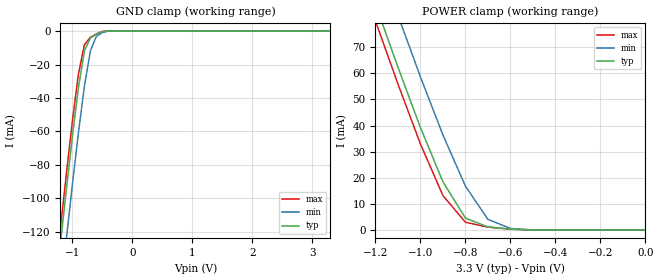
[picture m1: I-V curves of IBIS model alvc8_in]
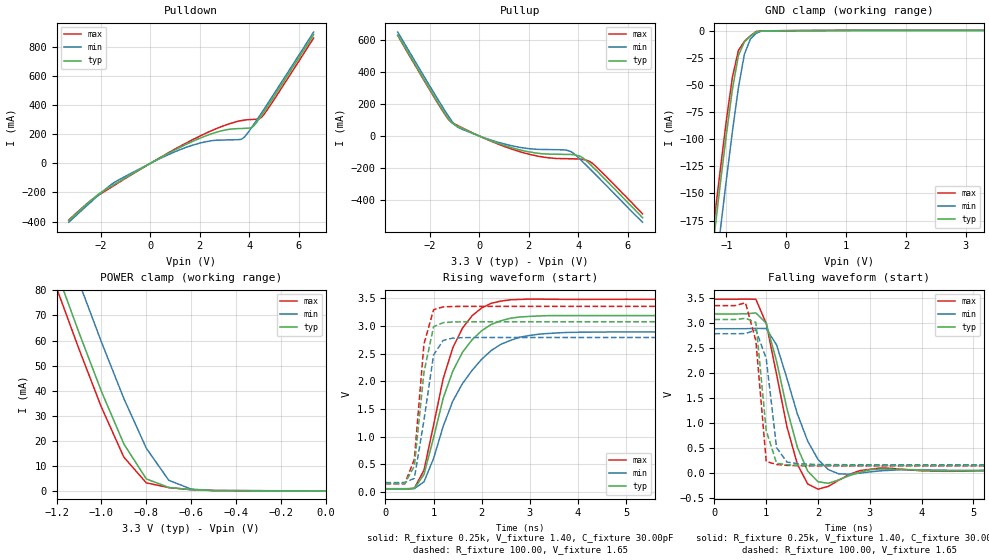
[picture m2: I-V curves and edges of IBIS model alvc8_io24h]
| IBIS file 16260ah.ibs created by s2ibis2 version 1.1
| North Carolina State University Electronics Research Laboratory  1995
[IBIS ver]   2.1
[File name]   16260ah.ibs
[File Rev]   1.0
[Date]   03/01/99 rtk rtk
[Source]   Integrated Device Technology, Inc.
[Notes]   1.Temperatures: typ=25C, min=100C, max=0C 2.RRmp rates based
   on 50 ohm load.
[Disclaimer] Integrated Device Technology, Inc. ("IDT") hereby grants the
   user of this IBIS model a non-exclusive, nontransferable
   license to use this IBIS model under the following terms. The
   user is granted this license only to use the IBIS model and is
   not granted rights to sell, copy (except as needed to run the
   IBIS model), rent, lease or sub-license the IBIS model in
   whole or in part, or in modified form to anyone. The User may
   modify the IBIS model to suit its specific applications, but
   rights to derivative works and such modifications shall belong
   to IDT. This IBIS model is provided on an AS IS" basis and IDT
   makes absolutely no warranty with respect to the information
   contained herein. IDT DISCLAIMS AND CUSTOMER WAIVES ALL
   WARRANTIES, EXPRESS AND IMPLIED, INCLUDING WARRANTIES OF
   MERCHANTABILITY AND FITNESS FOR A PARTICULAR PURPOSE. THE
   ENTIRE RISK AS TO QUALITY AND PERFORMANCE IS WITH THE USER
   ACCORDINGLY, IN NO EVENT SHALL IDT BE LIABLE FOR ANY DIRECT OR
   INDIRECT DAMAGES, WHETHER IN CONTRACT OR TORT, INCLUDING ANY
   LOST PROFITS OR OTHER INCIDENTAL, CONSEQUENTIAL, EXEMPLARY, OR
   PUNITIVE DAMAGES ARISING OUT OF THE USE OR APPLICATION OF THE
   IBIS model. Further, IDT reserves the right to make changes
   without notice to any product herein to improve reliability,
   function, or design. IDT does not convey any license under
   patent rights or any other intellectual property rights,
   including those of third parties. IDT is not obligated to
   provide maintenance or support for the licensed IBIS model.
[Copyright]   Copyright 1997, Integrated Device Technology, Inc. all rights
   reserved
|   Component ALVCH16260
[Component]   ALVCH1620
[Manufacturer]   Integrated Device Technology
[Package]
| PA56
| variable   typ   min   max
R_pkg   6.50m   5.00m   10.00m
L_pkg   3.30nH   2.50nH   4.90nH
C_pkg   0.29pF   0.010pF   1.16pF
[Pin]  signal_name   model_name   R_pin   L_pin   C_pin
1   OEA_   alvc8_in
2   LE1B   alvc8_in
3   2B3   alvc8_io24h
4   GND   GND
5   2B2   alvc8_io24h
6   2B1   alvc8_io24h
7   VCC   POWER
8   A1   alvc8_io24h
9   A2   alvc8_io24h
10   A3   alvc8_io24h
11   GND   GND
12   A4   alvc8_io24h
13   A5   alvc8_io24h
14   A6   alvc8_io24h
15   A7   alvc8_io24h
16   A8   alvc8_io24h
17   A9   alvc8_io24h
18   GND   GND
19   A10   alvc8_io24h
20   A11   alvc8_io24h
21   A12   alvc8_io24h
22   VCC   POWER
23   1B1   alvc8_io24h
24   1B2   alvc8_io24h
25   GND   alvc8_io24h
26   1B3   alvc8_io24h
27   LE2B   alvc8_in
28   SEL   alvc8_in
29   OE1B_   alvc8_in
30   LEA1B   alvc8_in
31   1B4   alvc8_io24h
32   GND   GND
33   1B5   alvc8_io24h
34   1B6   alvc8_io24h
35   VCC   POWER
36   1B7   alvc8_io24h
37   1B8   alvc8_io24h
38   1B9   alvc8_io24h
39   GND   GND
40   1B10   alvc8_io24h
41   1B11   alvc8_io24h
42   1B12   alvc8_io24h
43   2B12   alvc8_io24h
44   2B11   alvc8_io24h
45   2B10   alvc8_io24h
46   GND   GND
47   2B9   alvc8_io24h
48   2B8   alvc8_io24h
49   2B7   alvc8_io24h
50   VCC   POWER
51   2B6   alvc8_io24h
52   2B5   alvc8_io24h
53   GND   GND
54   2B4   alvc8_io24h
55   LEA2B   alvc8_in
56   OE2B_   alvc8_in
| Models and submodels in the file (2): alvc8_in (Input), alvc8_io24h (I/O)
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| in   in   dummy_model
| oe   oe   dummy_model
|   Model alvc8_in
[Model]   alvc8_in
Model_type   Input
Vinl =  0.800V
Vinh =  2.000V
C_comp   3.00pF   NA   NA
[Temperature Range]   25.00   100.00   0.000
[Voltage Range]   3.30V   3.00V   3.60V
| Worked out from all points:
|   GND clamp passes 1 mA (typ) near -0.54 V on its own axis
|   POWER clamp passes 1 mA (typ) near -0.68 V on its own axis
[GND_clamp]
| voltage   I(typ)   I(min)   I(max)
-3.3V     -860mA     -887mA     -851mA
-1.3V     -161mA     -190mA     -151mA
-1.2V     -127mA     -157mA     -118mA
-1.1V     -94.41mA   -124mA     -84.85mA
-1V       -62.78mA   -91.54mA   -53.52mA
-900mV    -33.71mA   -60.78mA   -25.6mA
-800mV    -11.74mA   -32.83mA   -8.09mA
-700mV    -4.033mA   -11.65mA   -3.7mA
-600mV    -1.899mA   -3.108mA   -1.699mA
-500mV    -308uA     -810uA     -172uA
-400mV    -3.848nA   -9.872uA   -399pA
3.3V      39.6pA     19.33nA    26.4pA
[POWER_clamp]
| voltage   I(typ)   I(min)   I(max)
-3.3V     630mA      648mA      624mA
-1.2V     86.56mA    106mA      80.02mA
-1.1V     62.33mA    82.22mA    55.88mA
-1V       39.2mA     58.61mA    32.91mA
-900mV    18.4mA     36.35mA    13.15mA
-800mV    4.556mA    16.76mA    2.954mA
-700mV    1.164mA    4.056mA    1.087mA
-600mV    320uA      578uA      299uA
-500mV    40.08nA    12.23uA    3.465nA
0V        39.6pA     59.11pA    43.2pA
|   Model alvc8_io24h
[Model]   alvc8_io24h
Model_type   I/O
Polarity   Non-Inverting
Enable   Active-High
Vinl =  0.000V
Vinh =  2.000V
Vmeas =  1.500V
C_comp   3.00pF   NA   NA
[Temperature Range]   25.00   100.00   0.000
[Voltage Range]   3.30V   3.00V   3.60V
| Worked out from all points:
|   slope of the pulldown table from 0 to 0.495 V, typ, clamps not added: 10.5 ohm
|   slope of the pullup table from 0 to 0.495 V, typ, clamps not added: 16.1 ohm
|   GND clamp passes 1 mA (typ) near -0.50 V on its own axis
|   POWER clamp passes 1 mA (typ) near -0.66 V on its own axis
|   rising waveform, R_fixture 0.25k, V_fixture 1.40, C_fixture 30.00pF: 20-80 % time 723ps typ, 920ps min, 623ps max; typ from 0.055 V to 3.19 V
|   rising waveform, R_fixture 100.00, V_fixture 1.65: 20-80 % time 248ps typ, 279ps min, 194ps max; typ from 0.155 V to 3.08 V
|   falling waveform, R_fixture 0.25k, V_fixture 1.40, C_fixture 30.00pF: 20-80 % time 444ps typ, 538ps min, 413ps max; typ from 3.19 V to 0.055 V
|   falling waveform, R_fixture 100.00, V_fixture 1.65: 20-80 % time 187ps typ, 176ps min, 171ps max; typ from 3.08 V to 0.155 V
[Pulldown]
| voltage   I(typ)   I(min)   I(max)
-3.3V     -392mA     -404mA     -389mA
-2.3V     -240mA     -249mA     -241mA
-1.5V     -149mA     -136mA     -156mA
300mV     28.8mA     25.5mA     30.3mA
1.4V      127mA      107mA      135mA
2.4V      199mA      153mA      219mA
3.6V      239mA      163mA      291mA
3.8V      240mA      180mA      297mA
4.2V      260mA      272mA      302mA
4.4V      306mA      322mA      306mA
4.6V      356mA      373mA      337mA
6.6V      883mA      901mA      860mA
[Pullup]
| voltage   I(typ)   I(min)   I(max)
-3.3V     630mA      649mA      628mA
-1.4V     142mA      160mA      137mA
-1.1V     80.6mA     90.7mA     83.6mA
-900mV    63mA       57.7mA     67.6mA
400mV     -25.1mA    -21.5mA    -27.4mA
1.6V      -85mA      -69.5mA    -95.9mA
2.6V      -111mA     -84mA      -132mA
3.4V      -115mA     -86.1mA    -141mA
3.7V      -115mA     -97.1mA    -142mA
4.1V      -128mA     -149mA     -144mA
4.5V      -179mA     -210mA     -162mA
6.6V      -510mA     -538mA     -486mA
[GND_clamp]
| voltage   I(typ)   I(min)   I(max)
-3.3V     -1.238A    -1.278A    -1.225A
-1.3V     -235mA     -278mA     -221mA
-1.2V     -187mA     -230mA     -173mA
-1.1V     -140mA     -183mA     -127mA
-1V       -95.39mA   -137mA     -82.2mA
-900mV    -54.08mA   -92.95mA   -42.96mA
-800mV    -22.96mA   -52.74mA   -18.28mA
-700mV    -10.43mA   -21.77mA   -9.816mA
-600mV    -5.251mA   -7.746mA   -4.745mA
-500mV    -1.015mA   -2.281mA   -688uA
-400mV    -144uA     -128uA     -169uA
3.3V      264uA      161uA      341uA
[POWER_clamp]
| voltage   I(typ)   I(min)   I(max)
-3.3V     638mA      656mA      632mA
-1.2V     87.67mA    108mA      81.05mA
-1.1V     63.19mA    83.28mA    56.62mA
-1V       39.75mA    59.43mA    33.41mA
-900mV    18.73mA    36.86mA    13.47mA
-800mV    4.8mA      17.05mA    3.222mA
-700mV    1.374mA    4.243mA    1.32mA
-600mV    498uA      728uA      497uA
-500mV    146uA      134uA      162uA
0V        111pA      156pA      121pA
[Ramp]
| variable   typ   min   max
dV/dt_r   1.48/0.31n   1.29/0.30n   1.66/0.22n
dV/dt_f   1.63/0.28n   1.45/0.31n   1.80/0.19n
R_load = 50.00
[Rising Waveform]
R_fixture = 0.25k
V_fixture = 1.40
C_fixture = 30.00pF
R_dut = 7.00m
L_dut = 3.30nH
C_dut = 0.29pF
| time   V(typ)   V(min)   V(max)
0s        55.43mV    62mV       53.03mV
600ps     66.6mV     63.52mV    70.73mV
800ps     318mV      185mV      393mV
1ns       982mV      608mV      1.211V
1.2ns     1.697V     1.189V     2.05V
1.4ns     2.186V     1.644V     2.606V
1.8ns     2.751V     2.198V     3.185V
2.4ns     3.095V     2.67V      3.451V
3.8ns     3.189V     2.885V     3.481V
19.8ns    3.189V     2.893V     3.482V
[Rising Waveform]
R_fixture = 100.00
V_fixture = 1.65
R_dut = 7.00m
L_dut = 3.30nH
C_dut = 0.29pF
| time   V(typ)   V(min)   V(max)
0s        155mV      172mV      148mV
400ps     155mV      173mV      148mV
600ps     469mV      249mV      594mV
800ps     2.166V     1.299V     2.675V
1ns       2.988V     2.477V     3.294V
1.2ns     3.061V     2.741V     3.346V
1.4ns     3.073V     2.782V     3.353V
2ns       3.077V     2.793V     3.355V
19.8ns    3.077V     2.793V     3.355V
[Falling Waveform]
R_fixture = 0.25k
V_fixture = 1.40
C_fixture = 30.00pF
R_dut = 7.00m
L_dut = 3.30nH
C_dut = 0.29pF
| time   V(typ)   V(min)   V(max)
0s        3.189V     2.893V     3.482V
800ps     3.208V     2.901V     3.481V
1ns       3.002V     2.896V     2.998V
1.2ns     2.239V     2.568V     1.977V
1.4ns     1.294V     1.899V     934mV
1.6ns     525mV      1.193V     186mV
2ns       -168mV     277mV      -316mV
2.4ns     -131mV     -10.2mV    -138mV
3.2ns     86.4mV     50.55mV    107mV
19.8ns    55.43mV    62mV       53.03mV
[Falling Waveform]
R_fixture = 100.00
V_fixture = 1.65
R_dut = 7.00m
L_dut = 3.30nH
C_dut = 0.29pF
| time   V(typ)   V(min)   V(max)
0s        3.077V     2.793V     3.355V
400ps     3.077V     2.793V     3.355V
600ps     3.101V     2.795V     3.411V
800ps     3.02V      2.869V     2.651V
1ns       857mV      2.294V     237mV
1.2ns     202mV      512mV      177mV
1.4ns     172mV      227mV      160mV
1.6ns     163mV      194mV      154mV
2ns       157mV      178mV      149mV
19.8ns    155mV      172mV      148mV
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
